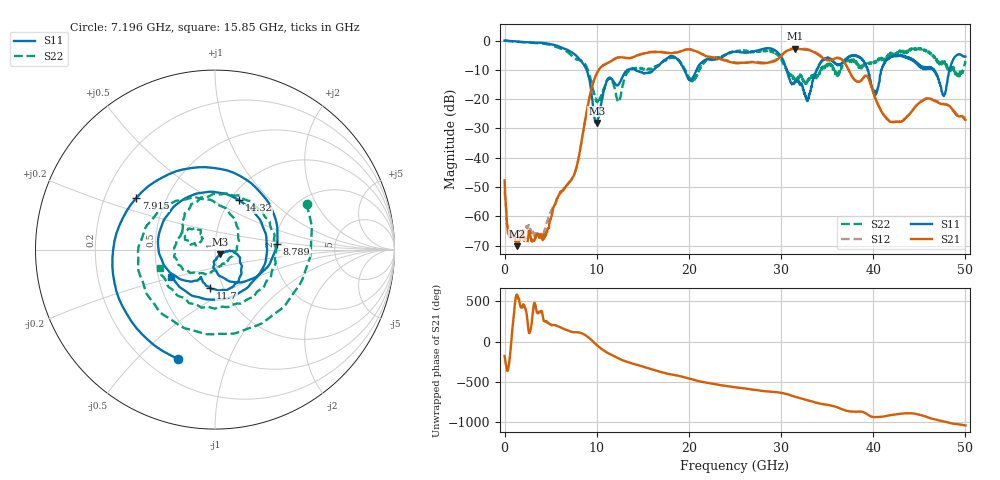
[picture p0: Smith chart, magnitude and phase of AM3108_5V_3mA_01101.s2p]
# Hz S DB R 50.0
!freq dBS11 angS11 dBS21 angS21 dBS12 angS12 dBS22 angS22
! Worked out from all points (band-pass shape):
!   1601 points, 10 MHz to 50 GHz, reference 50 ohm
!   highest |S21| = -2.75 dB at 31.53 GHz (marker M1); lowest = -70.2 dB at 1.385 GHz (marker M2)
!   |S21| within 3 dB of the highest: 13.87 GHz to 22.64 GHz (8.765 GHz wide, 48 % of centre); 29.86 GHz to 34.46 GHz (4.597 GHz wide, 14.3 % of centre)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
!   lowest |S11| = -28.1 dB at 10.01 GHz (marker M3), VSWR 1.08, Z = 53 - j2.67 ohm
!   |S11| at or under -10 dB: 8.91 GHz to 13.33 GHz (4.42 GHz wide, 39.8 % of centre); 14.2 GHz to 16.19 GHz (1.983 GHz wide, 13.1 % of centre); 30.62 GHz to 33.85 GHz (3.23 GHz wide, 10 % of centre)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
!   |S22| runs from -21.0 to 0.1 dB; largest |S21 - S12| = 0.024
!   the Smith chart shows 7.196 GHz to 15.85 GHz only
!   S11 on the Smith chart (normalised r, x): 7.196 GHz: 0.32, -0.67; 7.915 GHz: 0.34, +0.27; 8.789 GHz: 2.05, +0.15; 11.7 GHz: 0.87, -0.39; 14.32 GHz: 1.10, +0.67; 15.85 GHz: 0.59, -0.20
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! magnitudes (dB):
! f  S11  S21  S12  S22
! 10 MHz  0.0  -47.7  -51.5  0.1
! 541.1 MHz  -0.1  -66.9  -65.6  -0.2
! 1.385 GHz  -0.3  -70.2  -65.6  -0.4
! 4.384 GHz  -0.9  -67.0  -64.1  -1.1
! 7.196 GHz  -3.8  -47.7  -47.8  -4.9
! 7.915 GHz  -5.6  -41.9  -41.9  -6.5
! 8.352 GHz  -7.1  -34.5  -34.6  -6.9
! 8.789 GHz  -9.2  -26.4  -26.3  -8.3
! 10.01 GHz  -28.1  -11.2  -11.1  -20.3
! 11.7 GHz  -13.4  -6.7  -6.6  -13.7
! 14.32 GHz  -10.3  -5.1  -5.0  -9.6
! 15.85 GHz  -10.8  -3.9  -3.8  -9.9
! 16.69 GHz  -8.6  -3.9  -3.6  -8.6
! 25 GHz  -3.8  -7.7  -7.4  -3.7
! 29.16 GHz  -3.0  -7.2  -6.9  -3.7
! 31.53 GHz  -14.1  -2.7  -2.7  -13.8
! 33.35 GHz  -15.5  -3.6  -3.4  -12.7
! 38 GHz  -5.0  -13.5  -13.4  -6.6
! 40.22 GHz  -18.6  -19.7  -19.6  -7.6
! 41.69 GHz  -6.0  -27.3  -27.0  -5.2
! 47.66 GHz  -18.9  -21.7  -21.6  -7.7
! 50 GHz  -5.5  -27.1  -26.6  -6.9
